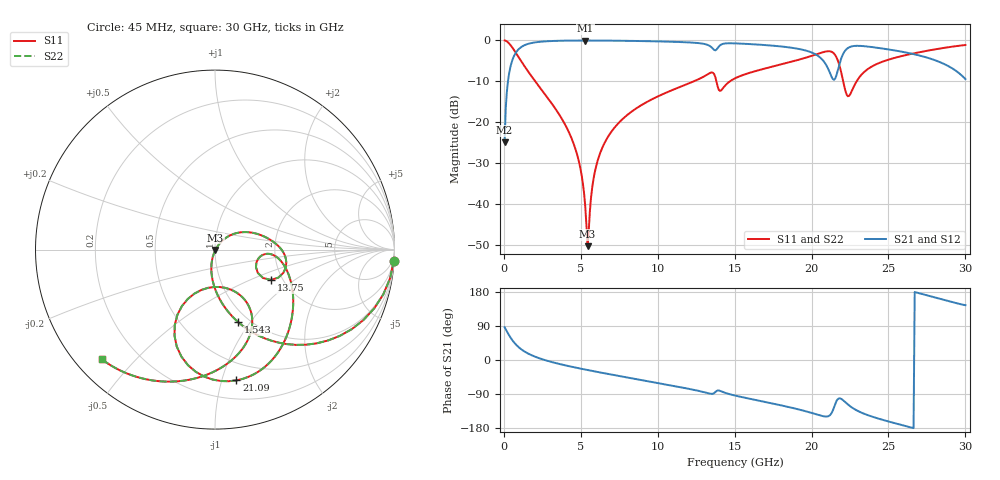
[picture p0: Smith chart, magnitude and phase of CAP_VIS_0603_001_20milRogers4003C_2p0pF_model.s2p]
! S-parameter model data by Modelithics Inc.  support@modelithics.com  813-866-6335  Tampa FL USA
! S-Parameter data specifications:
! Substrate: 20-mil Rogers 4003C, substrate thickness, H=0.508mm, Dielectric constant, Er=3.75
! PCB Mounting Pad Footprint: Pad width, PadW=0.90mm , Pad length, PadL=1.00mm , Pad gap, PadG (edge-to-edge)=1.00mm , Reference planes=3.0mm apart
! Created Wed Nov 18 13:19:39 2015
# hz S ma R 50
! 2 Port Network Data from SP1.SP block
! freq  magS11  angS11  magS21  angS21  magS12  angS12  magS22  angS22
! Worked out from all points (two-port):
!   401 points, 45 MHz to 30 GHz, reference 50 ohm
!   highest |S21| = -0.03 dB at 5.287 GHz (marker M1); lowest = -24.9 dB at 45 MHz (marker M2)
!   |S21| within 3 dB of the highest: 771.5 MHz to 20.06 GHz (19.28 GHz wide, 185 % of centre); 22.09 GHz to 26.24 GHz (4.145 GHz wide, 17.2 % of centre)
!   lowest |S11| = -50.2 dB at 5.437 GHz (marker M3), VSWR 1.01, Z = 50.2 - j0.19 ohm
!   |S11| at or under -10 dB: 2.04 GHz to 12.34 GHz (10.3 GHz wide, 143 % of centre); 13.82 GHz to 14.69 GHz (871.5 MHz wide, 6.12 % of centre); 22.06 GHz to 22.93 GHz (870.2 MHz wide, 3.87 % of centre)
!   |S22| runs from -50.2 to 0.0 dB; largest |S21 - S12| = 0
!   S11 on the Smith chart (normalised r, x): 45 MHz: 1, -33; 1.543 GHz: 0.89, -0.88; 13.75 GHz: 1.74, -0.67; 21.09 GHz: 0.35, -1.11; 30 GHz: 0.08, -0.40
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4.5e7  0.9984 -3.5  0.05705 86.5  0.05705 86.5  0.9984 -3.5
2.696625e8  0.9458 -20.3  0.3246 69.7  0.3246 69.7  0.9458 -20.3
4.94325e8  0.8448 -34.7  0.5345 55.2  0.5345 55.2  0.8448 -34.7
1.54275e9  0.4257 -72.1  0.9033 17.7  0.9033 17.7  0.4257 -72.1
4.088925e9  0.08554 -103.3  0.9934 -15.0  0.9934 -15.0  0.08554 -103.3
5.062462e9  0.0221 -105.9  0.9964 -23.4  0.9964 -23.4  0.0221 -105.9
5.287125e9  0.009448 -96.9  0.9965 -25.2  0.9965 -25.2  0.009448 -96.9
5.4369e9  0.003086 -37.9  0.9965 -26.5  0.9965 -26.5  0.003086 -37.9
5.961112e9  0.02738 52.7  0.9959 -30.6  0.9959 -30.6  0.02738 52.7
6.6351e9  0.0605 51.0  0.9942 -35.8  0.9942 -35.8  0.0605 51.0
1.007992e10  0.2104 27.4  0.9719 -61.3  0.9719 -61.3  0.2104 27.4
1.374941e10  0.3539 -28.5  0.7562 -84.3  0.7562 -84.3  0.3539 -28.5
1.412385e10  0.2458 -12.0  0.8895 -82.6  0.8895 -82.6  0.2458 -12.0
1.50225e10  0.3445 -6.7  0.92 -93.8  0.92 -93.8  0.3445 -6.7
2.003996e10  0.6504 -54.6  0.7076 -140.1  0.7076 -140.1  0.6504 -54.6
2.108839e10  0.7383 -80.7  0.4463 -148.3  0.4463 -148.3  0.7383 -80.7
2.176238e10  0.5301 -115.2  0.4747 -101.6  0.4747 -101.6  0.5301 -115.2
2.236148e10  0.2083 -91.2  0.8064 -117.3  0.8064 -117.3  0.2083 -91.2
2.333501e10  0.3977 -59.9  0.8525 -140.5  0.8525 -140.5  0.3977 -59.9
2.505742e10  0.5866 -76.3  0.7728 -162.9  0.7728 -162.9  0.5866 -76.3
2.782826e10  0.7659 -106.5  0.5903 167.2  0.5903 167.2  0.7659 -106.5
3e10  0.8781 -135.9  0.3378 144.6  0.3378 144.6  0.8781 -135.9
